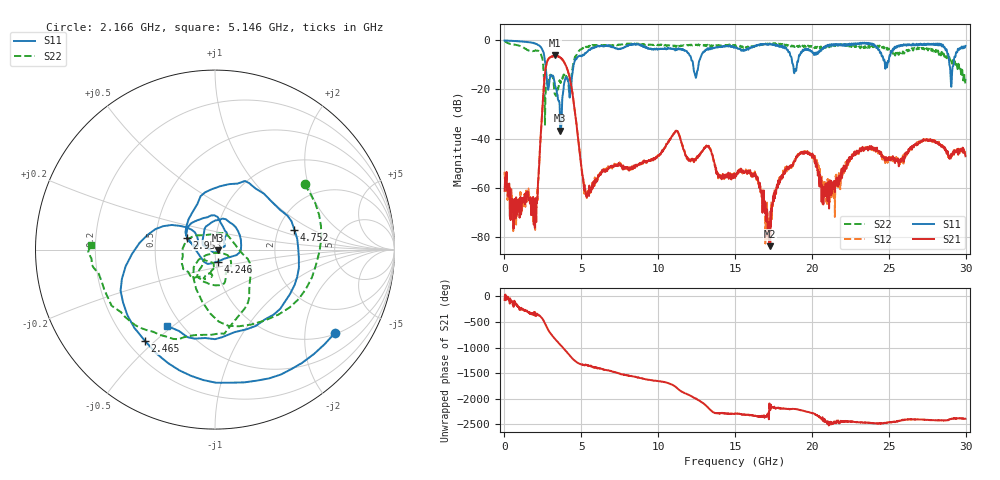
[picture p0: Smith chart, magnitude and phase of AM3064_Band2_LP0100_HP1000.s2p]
# Hz S DB R 50.0
!freq dBS11 angS11 dBS21 angS21 dBS12 angS12 dBS22 angS22
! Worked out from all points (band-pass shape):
!   1600 points, 10 MHz to 29.98 GHz, reference 50 ohm
!   highest |S21| = -6.14 dB at 3.271 GHz (marker M1); lowest = -83.9 dB at 17.29 GHz (marker M2)
!   |S21| within 3 dB of the highest: 2.753 GHz to 3.909 GHz (1.156 GHz wide, 34.7 % of centre)
!   lowest |S11| = -36.8 dB at 3.628 GHz (marker M3), VSWR 1.03, Z = 51.4 - j0.369 ohm
!   |S11| at or under -10 dB: 2.671 GHz to 4.499 GHz (1.828 GHz wide, 51 % of centre); 12.27 GHz to 12.62 GHz (346.3 MHz wide, 2.78 % of centre); 28.95 GHz to 29.2 GHz (256.8 MHz wide, 0.883 % of centre)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
!   |S22| runs from -34.7 to -0.2 dB; largest |S21 - S12| = 0.014
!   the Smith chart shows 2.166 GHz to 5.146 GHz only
!   S11 on the Smith chart (normalised r, x): 2.166 GHz: 1.03, -2.83; 2.465 GHz: 0.27, -0.46; 2.953 GHz: 0.73, +0.10; 4.246 GHz: 1.02, -0.14; 4.752 GHz: 2.45, +0.69; 5.146 GHz: 0.42, -0.48
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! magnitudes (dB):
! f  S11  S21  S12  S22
! 10 MHz  0.0  -61.3  -53.5  -0.2
! 703.5 MHz  -0.2  -65.3  -67.1  -1.8
! 2.166 GHz  -1.8  -62.1  -60.1  -4.2
! 2.465 GHz  -3.9  -27.6  -27.6  -7.3
! 2.953 GHz  -15.4  -7.0  -7.0  -14.2
! 3.271 GHz  -17.5  -6.1  -6.2  -21.8
! 3.628 GHz  -36.8  -7.0  -6.9  -17.1
! 4.246 GHz  -23.3  -15.3  -15.2  -19.8
! 4.752 GHz  -6.8  -38.1  -37.7  -5.1
! 5.015 GHz  -6.5  -52.1  -52.0  -3.7
! 5.146 GHz  -6.0  -58.5  -57.6  -3.2
! 10 GHz  -3.5  -46.8  -46.7  -1.8
! 11.18 GHz  -3.5  -37.0  -37.1  -2.6
! 12.44 GHz  -14.9  -48.7  -49.0  -1.9
! 15 GHz  -2.6  -56.1  -54.8  -2.0
! 16.32 GHz  -2.2  -55.1  -55.2  -2.2
! 17.29 GHz  -1.7  -83.9  -75.8  -1.3
! 18.17 GHz  -2.7  -53.6  -53.2  -2.2
! 19.99 GHz  -4.4  -47.4  -46.4  -2.3
! 20.83 GHz  -3.0  -60.1  -57.7  -2.6
! 25 GHz  -8.3  -48.6  -48.5  -3.3
! 29.98 GHz  -2.3  -47.2  -46.7  -15.7
